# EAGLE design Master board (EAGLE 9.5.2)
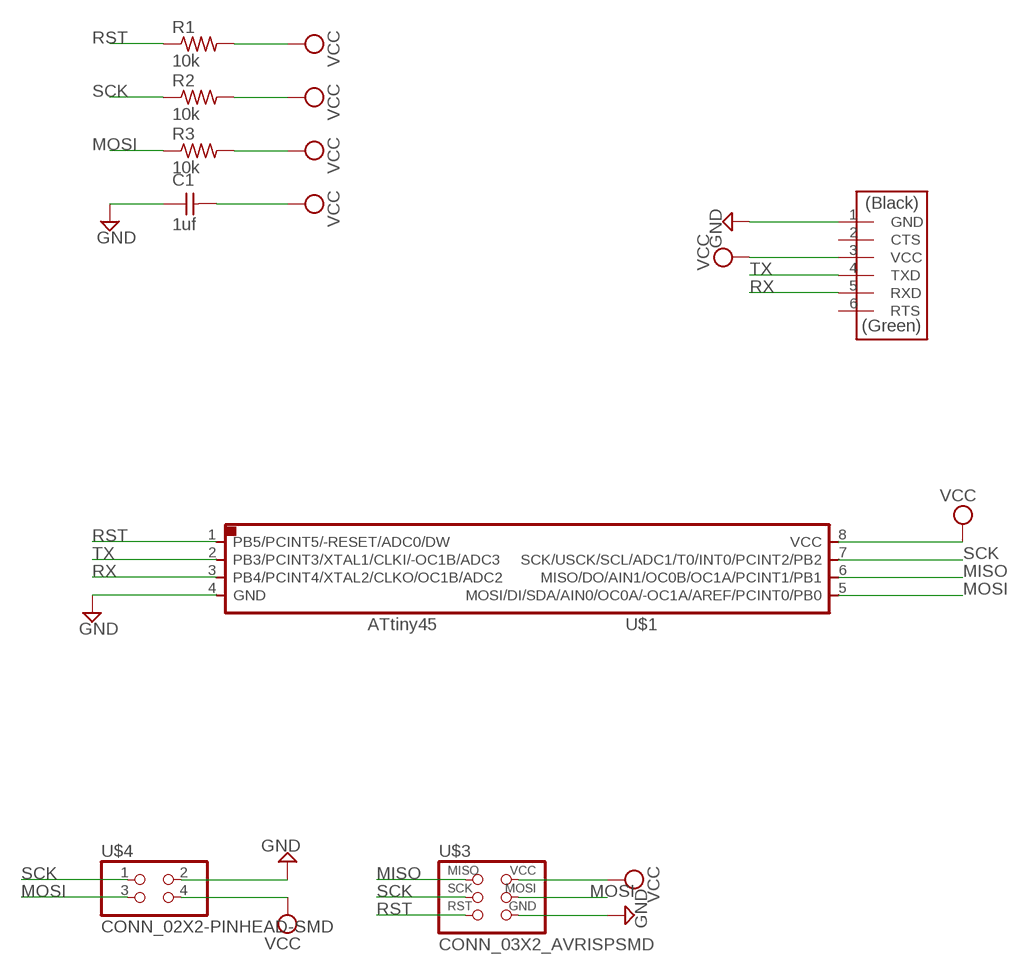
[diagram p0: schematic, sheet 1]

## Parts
C1  1uf  CAP_UNPOLARIZED  [C1206]
R1  10k  R1206  [R1206]
R2  10k  R1206  [R1206]
R3  10k  R1206  [R1206]
U$1  UC_ATTINY45SI  [SOIC8]
U$2  CONN_06_FTDI-SMD-HEADER  [1X06SMD]
U$3  CONN_03X2_AVRISPSMD  [2X03SMD]
U$4  CONN_02X2-PINHEAD-SMD  [2X02SMD]

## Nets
GND: C1.1 U$1.4(GND) U$2.1(GND) U$3.6(GND) U$4.2
MISO: U$1.6(MISO/DO/AIN1/OC0B/OC1A/PCINT1/PB1) U$3.1(MISO)
MOSI: R3.1 U$1.5(MOSI/DI/SDA/AIN0/OC0A/-OC1A/AREF/PCINT0/PB0) U$3.4(MOSI) U$4.3
RST: R1.1 U$1.1(PB5/PCINT5/-RESET/ADC0/DW) U$3.5(RST)
RX: U$1.3(PB4/PCINT4/XTAL2/CLKO/OC1B/ADC2) U$2.5(RXD)
SCK: R2.1 U$1.7(SCK/USCK/SCL/ADC1/T0/INT0/PCINT2/PB2) U$3.3(SCK) U$4.1
TX: U$1.2(PB3/PCINT3/XTAL1/CLKI/-OC1B/ADC3) U$2.4(TXD)
VCC: C1.2 R1.2 R2.2 R3.2 U$1.8(VCC) U$2.3(VCC) U$3.2(VCC) U$4.4
Unconnected: U$2.2(CTS) U$2.6(RTS)

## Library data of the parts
C1 = fab:CAP_UNPOLARIZED
R1-R3 = fab:R: Resistor (US Symbol)
U$1 = fab:UC_ATTINY45
U$2 = fab:CONN_06_FTDI-SMD-HEADER
U$3 = fab:CONN_03X2_AVRISP
U$4 = fab:CONN_02X2-PINHEAD-SMD

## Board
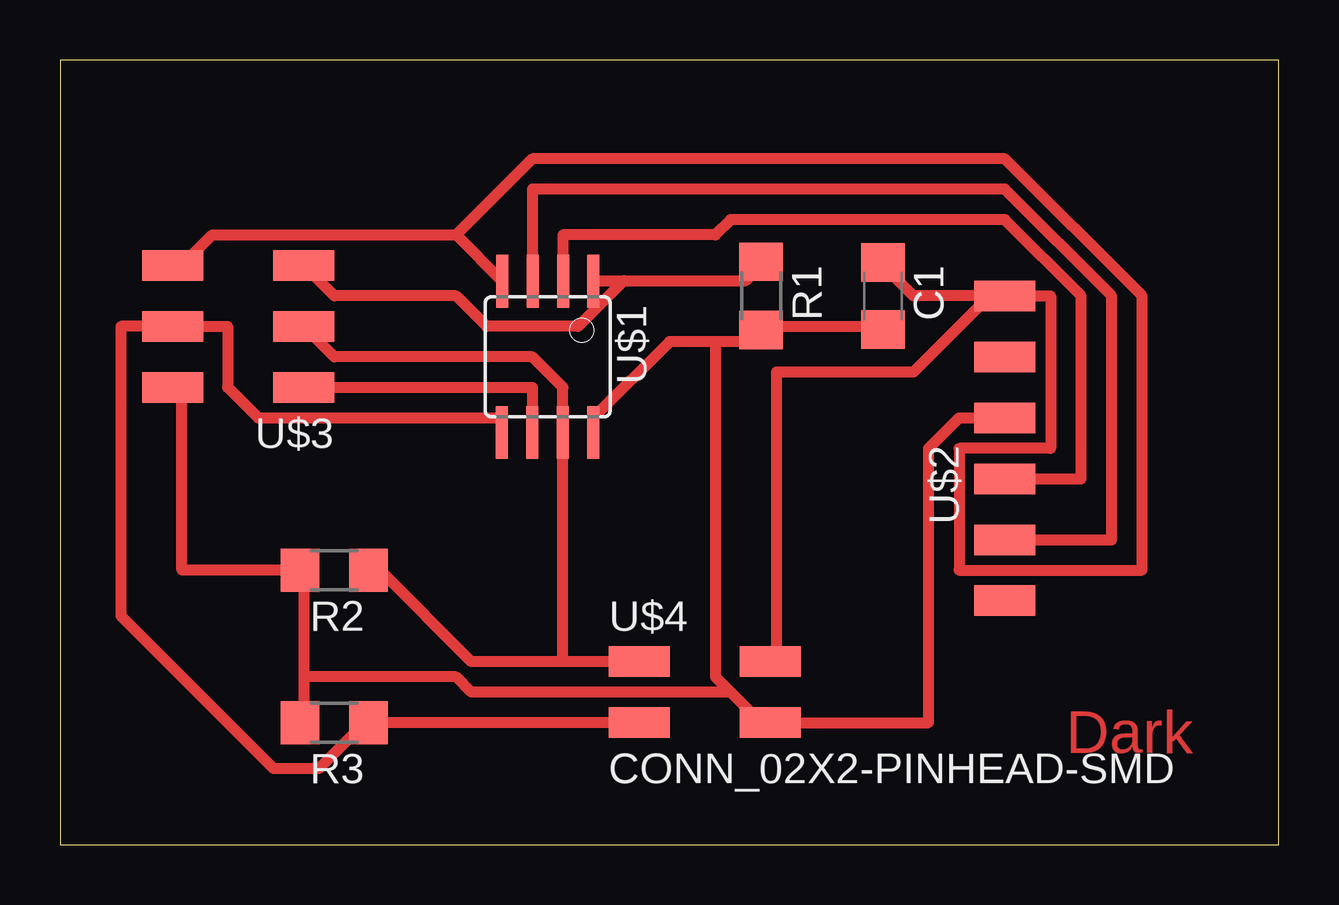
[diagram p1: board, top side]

Size 50.78 x 32.69 mm. Coordinates in mm from the lower left corner, seen from the top.
Outline: 0,0 50.78,0 50.78,32.69 0,32.69 0,0
Copper layers (1*16): Top 0.035mm / dielectric 1.5mm / Bottom 0.035mm
Design rules "fab-1": minimum track width 0.45mm, minimum drill 32mil, track to track 16mil, track to pad 16mil, pad to pad 16mil, via to via 16mil, smd to smd 6mil, copper to edge 16mil, drill to drill 16mil, minimum pad ring 10mil, minimum via ring 8mil, stop-mask expansion 4mil, vias tented up to drill 0mil, thermal gap 16mil

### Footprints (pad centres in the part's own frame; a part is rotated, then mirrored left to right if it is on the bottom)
C1206 = smd 1.6 x 1.8: 1 -1.4,0; 2 1.4,0
R1206 = smd 1.6 x 1.803: 1 -1.422,0; 2 1.422,0
SOIC8 = smd 0.5 x 2.2: 1 -1.905,-3.154; 2 -0.645,-3.154; 3 0.625,-3.154; 4 1.895,-3.154; 5 1.905,3.154; 6 0.635,3.154; 7 -0.635,3.154; 8 -1.905,3.154
1X06SMD = smd 2.54 x 1.27: 1 0,6.35; 2 0,3.81; 3 0,1.27; 4 0,-1.27; 5 0,-3.81; 6 0,-6.35
2X03SMD = smd 2.54 x 1.27: 1 -2.54,2.54; 2 2.92,2.54; 3 -2.54,0; 4 2.92,0; 5 -2.54,-2.54; 6 2.92,-2.54
2X02SMD = smd 2.54 x 1.27: 1 -2.54,1.27; 2 2.92,1.27; 3 -2.54,-1.27; 4 2.92,-1.27

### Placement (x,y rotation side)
C1  34.29,22.86 270 top
R1  29.21,22.86 270 top
R2  11.43,11.43 180 top
R3  11.43,5.08 180 top
U$1  20.32,20.32 180 top
U$2  39.37,16.51 0 top
U$3  7.62,21.59 180 top
U$4  26.67,6.35 0 top

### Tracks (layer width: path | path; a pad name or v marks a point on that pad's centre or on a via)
GND
  Top 0.45: 16.51,25.4 18.41,23.5 U$1.4 | 16.51,25.4 6.35,25.4 5.08,24.13 U$3.6 | 38.73,22.86 35.56,22.86 34.29,24.13 C1.1 | 38.73,22.86 35.56,19.68 29.85,19.68 29.85,7.62 U$4.2 | 38.73,22.86 U$2.1 41.28,22.86 41.28,16.51 37.47,16.51 37.47,11.43 45.09,11.43 45.09,22.86 39.37,28.57 19.69,28.57 16.51,25.4
MISO
  Top 0.45: U$1.6 19.69,19.05 U$3.1
MOSI
  Top 0.45: U$4.3 R3.1 12.7,5.08 10.8,3.17 8.89,3.17 2.54,9.52 2.54,21.59 U$3.4 6.98,21.59 6.98,19.05 8.26,17.78 18.41,17.78 U$1.5
RST
  Top 0.45: 23.5,23.5 22.23,23.5 U$1.1 | 23.5,23.5 28.58,23.5 29.21,24.13 R1.1 | U$3.5 11.43,22.86 16.51,22.86 17.78,21.59 21.59,21.59 23.5,23.5
RX
  Top 0.45: U$2.5 43.82,12.7 43.82,22.86 39.37,27.3 19.69,27.3 19.69,23.5 U$1.3
SCK
  Top 0.45: U$4.1 20.96,7.62 | 20.96,7.62 17.15,7.62 13.34,11.43 R2.1 | 20.96,7.62 U$1.7 20.96,19.05 19.69,20.32 11.43,20.32 U$3.3
TX
  Top 0.45: U$2.4 42.55,15.24 42.55,22.86 39.37,26.04 27.94,26.04 27.31,25.4 20.96,25.4 20.96,23.5 U$1.2
VCC
  Top 0.45: 10.16,6.98 10.16,11.43 R2.2 5.08,11.43 5.08,19.05 U$3.2 | 10.16,6.98 10.16,5.08 R3.2 | C1.2 34.29,21.59 29.21,21.59 R1.2 29.21,20.96 27.31,20.96 | 27.31,20.96 25.4,20.96 22.23,17.78 U$1.8 | 27.94,6.35 27.31,6.98 27.31,20.96 | 27.94,6.35 29.21,5.08 U$4.4 36.2,5.08 36.2,16.51 37.47,17.78 U$2.3 | 10.16,6.98 16.51,6.98 17.15,6.35 27.94,6.35

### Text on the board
Top: Dark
